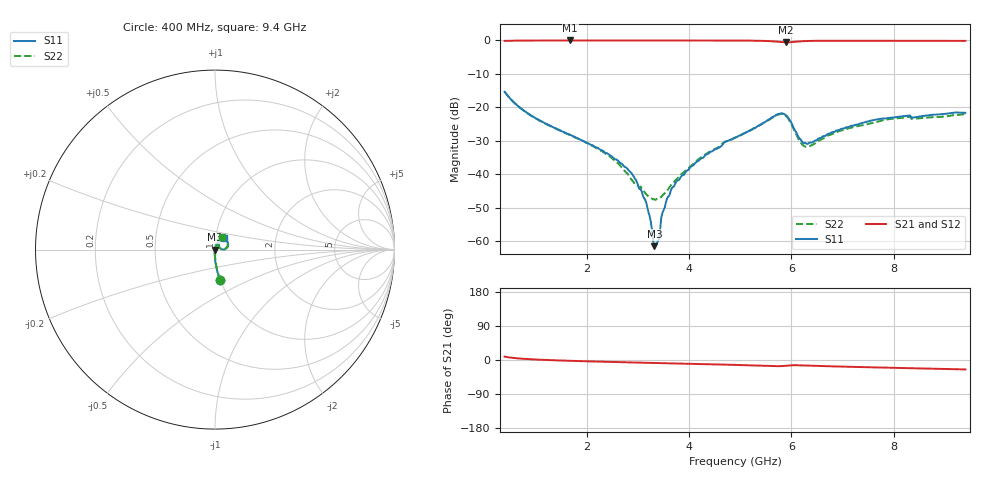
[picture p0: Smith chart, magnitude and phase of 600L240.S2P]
!  American Technical Ceramics  Date:  6/18/2004
!  One Norden Lane
!  Huntington Station,  NY.  11746-2102
!  Tel:  (631) 622-4700  Fax:  (631) 622-4748
!  Part Number  600L240  Mounting Orientation: Vertical
!  Description: Ultra Low ESR Microwave capacitors
!  Application: Coupling, Bypass, Tuning, DC Block
!  Filters, Matching
# GHZ S DB R 50
! Freq  |S11|  S11 Ph  |S21|  S21 Ph  |S12|  S12 Ph  |S22|  S22 Ph
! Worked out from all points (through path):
!   401 points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, 400 MHz to 9.4 GHz, reference 50 ohm
!   highest |S21| = -0.01 dB at 1.683 GHz (marker M1); lowest = -0.6 dB at 5.89 GHz (marker M2)
!   group delay of S21, straight-line fit = 8.47 ps
!   lowest |S11| = -61.5 dB at 3.325 GHz (marker M3), VSWR 1.00, Z = 49.9 - j0.0496 ohm
!   |S11| at or under -10 dB: start of sweep to end of sweep
!   |S22| runs from -47.6 to -15.3 dB; largest |S21 - S12| = 0.0036
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0.4  -15.35 -80.7  -0.14 8.8  -0.14 8.8  -15.34 -80.4
0.895  -22.21 -87.1  -0.03 2.1  -0.03 2.0  -22.27 -86.5
1.683  -28.19 -92.0  -0.01 -2.2  -0.01 -2.3  -28.36 -89.2
1.908  -29.85 -92.7  -0.01 -3.1  -0.01 -3.1  -29.88 -88.7
2.47  -34.48 -94.7  -0.01 -5.1  -0.01 -5.2  -34.87 -86.2
2.898  -40.05 -103.1  -0.02 -6.5  -0.02 -6.6  -41.97 -68.2
3.168  -48.60 -116.9  -0.01 -7.4  -0.01 -7.5  -45.94 -48.0
3.213  -51.46 -116.7  -0.01 -7.5  -0.02 -7.6  -46.59 -38.2
3.325  -61.46 -144.0  -0.02 -7.9  -0.02 -8.0  -47.48 -11.9
3.37  -60.60 159.5  -0.02 -8.1  -0.02 -8.2  -47.36 -3.0
3.415  -59.20 115.7  -0.02 -8.2  -0.02 -8.3  -47.18 5.9
3.528  -49.90 94.8  -0.02 -8.5  -0.01 -8.7  -45.67 29.8
3.73  -42.93 84.9  -0.02 -9.2  -0.02 -9.3  -41.86 51.5
4.18  -36.05 79.2  -0.03 -10.6  -0.03 -10.7  -35.55 69.6
4.9  -29.06 70.7  -0.04 -12.9  -0.05 -13.1  -29.08 69.0
5.71  -22.20 44.0  -0.36 -16.3  -0.38 -16.4  -22.38 46.1
5.89  -22.26 17.4  -0.58 -15.2  -0.61 -15.2  -22.52 19.4
6.205  -30.14 13.1  -0.23 -14.2  -0.25 -14.0  -30.99 17.6
6.408  -30.52 41.6  -0.13 -15.1  -0.13 -15.0  -31.26 49.3
6.948  -26.67 60.4  -0.07 -17.3  -0.06 -17.3  -27.01 68.7
7.915  -23.15 58.8  -0.07 -20.4  -0.07 -20.5  -23.51 69.4
9.4  -21.62 52.9  -0.13 -24.9  -0.14 -24.9  -21.96 59.2
